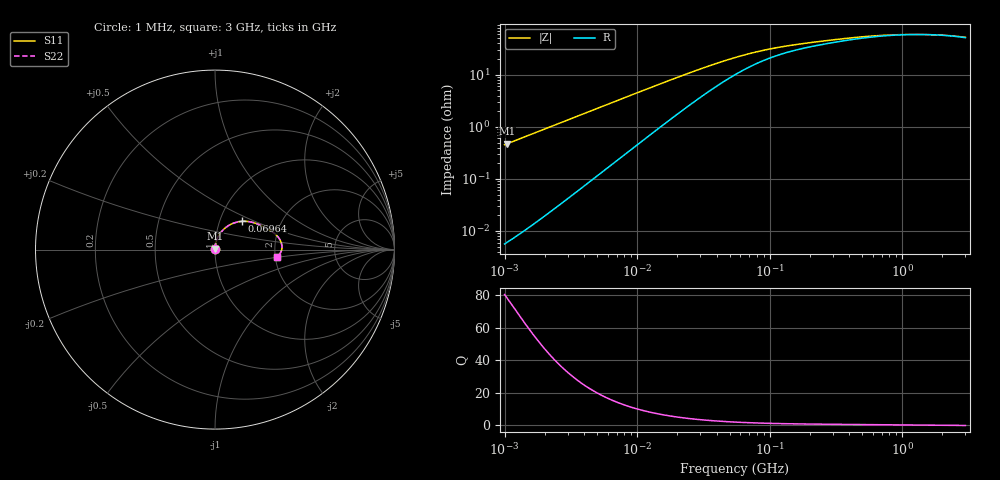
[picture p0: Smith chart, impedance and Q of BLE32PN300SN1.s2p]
! BLE32PN300SN1
# Hz S RI R 50
!Freq.(Hz) S11(Real) S11(Imag) S21(Real) S21(Imag) S12(Real) S12(Imag) S22(Real) S22(Imag)
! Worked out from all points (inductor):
!   401 points, 1 MHz to 3 GHz, reference 50 ohm
!   read as one part in series: L = 72.2 nH near 1.041 MHz
!   highest Q = 78.4 at 1.041 MHz (marker M1), where L = 72.3 nH
!   self-resonance near 1.552 GHz
!   S11 on the Smith chart (normalised r, x): 1 MHz: 1.00, +0.01; 69.64 MHz: 1.28, +0.42; 3 GHz: 2.03, -0.19
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1000000  7.7e-05 0.00454  0.9999 -0.00454  0.9999 -0.00454  7.7e-05 0.00454
1040844  8.25e-05 0.00472  0.9999 -0.00472  0.9999 -0.00472  8.25e-05 0.00472
3823119  0.000973 0.0173  0.999 -0.0173  0.999 -0.0173  0.000973 0.0173
7858845  0.00403 0.0352  0.996 -0.0352  0.996 -0.0352  0.00403 0.0352
1.461624e7  0.0135 0.0634  0.9865 -0.0634  0.9865 -0.0634  0.0135 0.0634
2.181181e7  0.0283 0.0897  0.9717 -0.0897  0.9717 -0.0897  0.0283 0.0897
3.065274e7  0.051 0.1155  0.949 -0.1155  0.949 -0.1155  0.051 0.1155
4.138676e7  0.0811 0.1372  0.9189 -0.1372  0.9189 -0.1372  0.0811 0.1372
5.477226e7  0.1173 0.1519  0.8827 -0.1519  0.8827 -0.1519  0.1173 0.1519
6.964249e7  0.1518 0.1576  0.8482 -0.1576  0.8482 -0.1576  0.1518 0.1576
8.854986e7  0.1862 0.1562  0.8138 -0.1562  0.8138 -0.1562  0.1862 0.1562
1.125904e8  0.2176 0.1494  0.7824 -0.1494  0.7824 -0.1494  0.2176 0.1494
1.49005e8  0.2489 0.1378  0.7511 -0.1378  0.7511 -0.1378  0.2489 0.1378
2.094008e8  0.2807 0.1224  0.7193 -0.1224  0.7193 -0.1224  0.2807 0.1224
3.124888e8  0.3131 0.1038  0.6869 -0.1038  0.6869 -0.1038  0.3131 0.1038
4.391493e8  0.3374 0.0853  0.6626 -0.0853  0.6626 -0.0853  0.3374 0.0853
5.929311e8  0.3545 0.0663  0.6455 -0.0663  0.6455 -0.0663  0.3545 0.0663
8.005644e8  0.3663 0.0457  0.6337 -0.0457  0.6337 -0.0457  0.3663 0.0457
1.147801e9  0.3727 0.0206  0.6273 -0.0206  0.6273 -0.0206  0.3727 0.0206
1.645649e9  0.3708 -0.00391  0.6292 0.00391  0.6292 0.00391  0.3708 -0.00391
2.221924e9  0.3617 -0.0234  0.6383 0.0234  0.6383 0.0234  0.3617 -0.0234
3e9  0.3431 -0.0405  0.6569 0.0405  0.6569 0.0405  0.3431 -0.0405
